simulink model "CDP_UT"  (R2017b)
settings: Solver=FixedStepDiscrete  StartTime=0.0  StopTime=10.0  FixedStep=0.01  RelTol=1e-3  EnableMultiTasking=on
undefined symbols (not defined in the file): ASWTYPE_FALSE, ASWTYPE_TRUE, CaCDP_CellTempNTCVoltTable_mV, CaCDP_CellTempTable_C, CaCDP_CMUPCBTempNTCVoltTable_mV, CaCDP_CMUPCBTempTable_C, CbCDP_DiffBusbarTempStateCheck_flg, CbCDP_DiffCellTempStateCheck_flg, CbCDP_DiffCellVoltStateCheck_flg, CbCDP_IgnorUpdateVld_flg, CbCDP_MaxBusbarTempStateCheck_flg, CbCDP_MaxCellTempStateCheck_flg, CbCDP_MaxCellVoltStateCheck_flg, CbCDP_MinBusbarTempStateCheck_flg, CbCDP_MinCellTempStateCheck_flg, CbCDP_MinCellVoltStateCheck_flg, CcCDP_AFETempConfig_numb, CcCDP_AFETempFltThd_C, CcCDP_AFETempFltThdHys_C, CcCDP_BusbarTempRngFltHiThrd_C, CcCDP_BusbarTempRngFltLowThrd_C, CcCDP_CellDiffFltLevel1_mV, CcCDP_CellDiffFltLevel2_mV, CcCDP_CellDiffFltLevel3_mV, CcCDP_CellTempLowerLimit_C, CcCDP_CellTempRngFltHiThrd_C, CcCDP_CellTempRngFltLowThrd_C, CcCDP_CellTempUpperLimit_C, CcCDP_CellVoltConfig_numb, CcCDP_CellVoltLowerLimit_mV, CcCDP_CellVoltRngHiThrd_mV, CcCDP_CellVoltRngLowThrd_mV, CcCDP_CellVoltUpdateThrd_numb, CcCDP_CellVoltUpperLimit_mV, CcCDP_ChrgMaxCellTempFltLv1Thrd_C, CcCDP_ChrgMaxCellTempFltLv2Thrd_C, CcCDP_ChrgMaxCellTempFltLv3Thrd_C, CcCDP_ChrgMaxCellTempReturnDiff_C, CcCDP_ChrgMinCellTempFltLv1Thrd_C, CcCDP_ChrgMinCellTempFltLv2Thrd_C, CcCDP_ChrgMinCellTempFltLv3Thrd_C, CcCDP_ChrgMinCellTempReturnDiff_C, CcCDP_CMUPCBTempConfig_numb, CcCDP_CMUPCBTempFltThd_C, CcCDP_CMUPCBTempFltThdHys_C, CcCDP_DiffBusbarTempFltLevel1Thrd_C, CcCDP_DiffBusbarTempFltLevel2Thrd_C, CcCDP_DiffBusbarTempReturnDifference_C, CcCDP_DiffCellTempFltLevel1Thrd_C, CcCDP_DiffCellTempFltLevel2Thrd_C, CcCDP_DiffCellTempReturnDifference_C, CcCDP_DiffCellVoltReturnDifference_mV, CcCDP_DiffVoltCheckMaxCellTempCondition_C, CcCDP_DiffVoltCheckMaxCellVoltCondition_mV, CcCDP_DiffVoltCheckMinCellTempCondition_C, CcCDP_DiffVoltCheckMinCellVoltCondition_mV, CcCDP_DiffVoltCheckPackCurrCondition_A, CcCDP_MaxAFETempIniVal_C, CcCDP_MaxBusbarTempFltLevel1Thrd_C, CcCDP_MaxBusbarTempFltLevel2Thrd_C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
libraries: AIWAYS_Powertrain_BMS_lib x148, simulink x8
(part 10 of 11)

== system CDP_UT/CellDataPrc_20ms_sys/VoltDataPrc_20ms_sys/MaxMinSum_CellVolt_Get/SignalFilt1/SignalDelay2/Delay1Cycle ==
  u : Inport
  Constant2 : Constant  Value=ASWTYPE_FALSE
  Switch : Switch  Criteria=u2 ~= 0  Threshold=1  RndMeth=Zero
  Unit Delay1 : UnitDelay  SampleTime=-1  StateName=StateName
  Unit Delay21 : UnitDelay  InitialCondition=1  SampleTime=-1  StateName=StateName
  y : Outport
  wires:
  Switch/1 -> y/1
  u/1 -> Switch/1, Unit Delay1/1
  Unit Delay1/1 -> Switch/3
  Unit Delay21/1 -> Switch/2
  Constant2/1 -> Unit Delay21/1

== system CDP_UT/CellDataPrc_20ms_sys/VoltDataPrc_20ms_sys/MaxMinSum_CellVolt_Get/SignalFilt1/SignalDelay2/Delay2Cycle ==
  u : Inport
  Constant2 : Constant  Value=ASWTYPE_FALSE
  Switch : Switch  Criteria=u2 ~= 0  Threshold=1  RndMeth=Zero
  Unit Delay1 : UnitDelay  SampleTime=-1  StateName=StateName
  Unit Delay2 : UnitDelay  InitialCondition=1  SampleTime=-1  StateName=StateName
  Unit Delay21 : UnitDelay  InitialCondition=1  SampleTime=-1  StateName=StateName
  Unit Delay3 : UnitDelay  SampleTime=-1  StateName=StateName
  y : Outport
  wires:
  Unit Delay3/1 -> Switch/3
  Unit Delay2/1 -> Switch/2
  Constant2/1 -> Unit Delay21/1
  Unit Delay21/1 -> Unit Delay2/1
  Unit Delay1/1 -> Unit Delay3/1
  u/1 -> Unit Delay1/1, Switch/1
  Switch/1 -> y/1

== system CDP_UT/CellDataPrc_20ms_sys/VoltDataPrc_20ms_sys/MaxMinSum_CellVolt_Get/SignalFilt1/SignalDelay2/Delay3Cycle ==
  u : Inport
  Constant2 : Constant  Value=ASWTYPE_FALSE
  Switch : Switch  Criteria=u2 ~= 0  Threshold=1  RndMeth=Zero
  Unit Delay1 : UnitDelay  SampleTime=-1  StateName=StateName
  Unit Delay2 : UnitDelay  InitialCondition=1  SampleTime=-1  StateName=StateName
  Unit Delay21 : UnitDelay  InitialCondition=1  SampleTime=-1  StateName=StateName
  Unit Delay3 : UnitDelay  SampleTime=-1  StateName=StateName
  Unit Delay4 : UnitDelay  InitialCondition=1  SampleTime=-1  StateName=StateName
  Unit Delay5 : UnitDelay  SampleTime=-1  StateName=StateName
  y : Outport
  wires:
  Unit Delay5/1 -> Switch/3
  Unit Delay4/1 -> Switch/2
  Unit Delay3/1 -> Unit Delay5/1
  Unit Delay2/1 -> Unit Delay4/1
  Constant2/1 -> Unit Delay21/1
  Unit Delay21/1 -> Unit Delay2/1
  Unit Delay1/1 -> Unit Delay3/1
  u/1 -> Unit Delay1/1, Switch/1
  Switch/1 -> y/1

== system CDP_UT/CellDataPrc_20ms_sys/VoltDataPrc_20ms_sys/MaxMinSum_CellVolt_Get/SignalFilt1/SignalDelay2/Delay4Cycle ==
  u : Inport
  Constant2 : Constant  Value=ASWTYPE_FALSE
  Switch : Switch  Criteria=u2 ~= 0  Threshold=1  RndMeth=Zero
  Unit Delay{1,3,5,7} (4 alike) : UnitDelay  SampleTime=-1  StateName=StateName
  Unit Delay{2,4,6,21} (4 alike) : UnitDelay  InitialCondition=1  SampleTime=-1  StateName=StateName
  y : Outport
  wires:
  Unit Delay7/1 -> Switch/3
  Unit Delay6/1 -> Switch/2
  Unit Delay5/1 -> Unit Delay7/1
  Unit Delay4/1 -> Unit Delay6/1
  Unit Delay3/1 -> Unit Delay5/1
  Unit Delay2/1 -> Unit Delay4/1
  Constant2/1 -> Unit Delay21/1
  Unit Delay21/1 -> Unit Delay2/1
  Unit Delay1/1 -> Unit Delay3/1
  u/1 -> Unit Delay1/1, Switch/1
  Switch/1 -> y/1

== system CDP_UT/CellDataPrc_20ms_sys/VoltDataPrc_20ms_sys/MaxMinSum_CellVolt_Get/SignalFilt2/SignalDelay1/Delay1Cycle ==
  u : Inport
  Constant2 : Constant  Value=ASWTYPE_FALSE
  Switch : Switch  Criteria=u2 ~= 0  Threshold=1  RndMeth=Zero
  Unit Delay1 : UnitDelay  SampleTime=-1  StateName=StateName
  Unit Delay21 : UnitDelay  InitialCondition=1  SampleTime=-1  StateName=StateName
  y : Outport
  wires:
  Constant2/1 -> Unit Delay21/1
  Unit Delay21/1 -> Switch/2
  Unit Delay1/1 -> Switch/3
  u/1 -> Unit Delay1/1, Switch/1
  Switch/1 -> y/1

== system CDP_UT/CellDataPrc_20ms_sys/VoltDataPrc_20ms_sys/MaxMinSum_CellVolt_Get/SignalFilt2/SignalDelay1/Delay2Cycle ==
  u : Inport
  Constant2 : Constant  Value=ASWTYPE_FALSE
  Switch : Switch  Criteria=u2 ~= 0  Threshold=1  RndMeth=Zero
  Unit Delay1 : UnitDelay  SampleTime=-1  StateName=StateName
  Unit Delay2 : UnitDelay  InitialCondition=1  SampleTime=-1  StateName=StateName
  Unit Delay21 : UnitDelay  InitialCondition=1  SampleTime=-1  StateName=StateName
  Unit Delay3 : UnitDelay  SampleTime=-1  StateName=StateName
  y : Outport
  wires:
  Switch/1 -> y/1
  u/1 -> Switch/1, Unit Delay1/1
  Unit Delay1/1 -> Unit Delay3/1
  Unit Delay21/1 -> Unit Delay2/1
  Constant2/1 -> Unit Delay21/1
  Unit Delay2/1 -> Switch/2
  Unit Delay3/1 -> Switch/3

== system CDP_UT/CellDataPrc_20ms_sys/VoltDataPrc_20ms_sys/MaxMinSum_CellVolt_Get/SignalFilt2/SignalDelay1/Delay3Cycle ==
  u : Inport
  Constant2 : Constant  Value=ASWTYPE_FALSE
  Switch : Switch  Criteria=u2 ~= 0  Threshold=1  RndMeth=Zero
  Unit Delay1 : UnitDelay  SampleTime=-1  StateName=StateName
  Unit Delay2 : UnitDelay  InitialCondition=1  SampleTime=-1  StateName=StateName
  Unit Delay21 : UnitDelay  InitialCondition=1  SampleTime=-1  StateName=StateName
  Unit Delay3 : UnitDelay  SampleTime=-1  StateName=StateName
  Unit Delay4 : UnitDelay  InitialCondition=1  SampleTime=-1  StateName=StateName
  Unit Delay5 : UnitDelay  SampleTime=-1  StateName=StateName
  y : Outport
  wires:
  Switch/1 -> y/1
  u/1 -> Switch/1, Unit Delay1/1
  Unit Delay1/1 -> Unit Delay3/1
  Unit Delay21/1 -> Unit Delay2/1
  Constant2/1 -> Unit Delay21/1
  Unit Delay2/1 -> Unit Delay4/1
  Unit Delay3/1 -> Unit Delay5/1
  Unit Delay4/1 -> Switch/2
  Unit Delay5/1 -> Switch/3

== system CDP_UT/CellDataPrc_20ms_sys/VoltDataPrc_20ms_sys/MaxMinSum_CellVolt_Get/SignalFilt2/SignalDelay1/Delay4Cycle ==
  u : Inport
  Constant2 : Constant  Value=ASWTYPE_FALSE
  Switch : Switch  Criteria=u2 ~= 0  Threshold=1  RndMeth=Zero
  Unit Delay{1,3,5,7} (4 alike) : UnitDelay  SampleTime=-1  StateName=StateName
  Unit Delay{2,4,6,21} (4 alike) : UnitDelay  InitialCondition=1  SampleTime=-1  StateName=StateName
  y : Outport
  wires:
  Switch/1 -> y/1
  u/1 -> Switch/1, Unit Delay1/1
  Unit Delay1/1 -> Unit Delay3/1
  Unit Delay21/1 -> Unit Delay2/1
  Constant2/1 -> Unit Delay21/1
  Unit Delay2/1 -> Unit Delay4/1
  Unit Delay3/1 -> Unit Delay5/1
  Unit Delay4/1 -> Unit Delay6/1
  Unit Delay5/1 -> Unit Delay7/1
  Unit Delay6/1 -> Switch/2
  Unit Delay7/1 -> Switch/3

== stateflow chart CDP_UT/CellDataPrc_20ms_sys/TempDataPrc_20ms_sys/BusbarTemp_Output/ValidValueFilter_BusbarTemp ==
  state VldValueFilter
    (default) -> (junction 1369)
    VldValueFilter -> (junction 1369)
    (junction 1369) -> (junction 1371) : {i = 0;}
    (junction 1373) -> (junction 1375) : [i < NumbConfig]
    (junction 1371) -> (junction 1373) : [i < InputNumb]
    (junction 1373) -> (junction 1377) : {OutputValue[i] = CcCDP_TempDefVal_C;}
    (junction 1375) -> (junction 1380) : {OutputValue[i] = InputValue[i];}
    (junction 1377) -> (junction 1371) : {i = i + 1;}
    (junction 1371) -> (junction 1385)
    (junction 1380) -> (junction 1377)
  (default) -> VldValueFilter
  data: InputValue input single; NumbConfig input uint8; i local uint8; CcCDP_TempDefVal_C parameter; OutputValue output single; InputNumb input uint8

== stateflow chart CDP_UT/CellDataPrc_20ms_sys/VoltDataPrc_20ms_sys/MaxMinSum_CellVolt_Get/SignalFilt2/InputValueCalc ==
  state VldValueFilter
    state Default
      Output_Value[0] = Input_Value;
      Output_Value[1] = Input_Value;
      Output_Value[2] = Input_Value;
      Output_Value[3] = Input_Value;
      Output_Value[4] = Input_Value;
    state NotUpdate
      Output_Value[0] = Old_Value[0];
      Output_Value[1] = Old_Value[1];
      Output_Value[2] = Old_Value[2];
      Output_Value[3] = Old_Value[3];
      Output_Value[4] = Old_Value[4];
    state Update
      Output_Value[0] = Input_Value;
      Output_Value[1] = Old_Value[0];
      Output_Value[2] = Old_Value[1];
      Output_Value[3] = Old_Value[2];
      Output_Value[4] = Old_Value[3];
    (default) -> Default
    VldValueFilter -> (junction 1397)
    (junction 1397) -> (junction 1398) : [Rige]
    (junction 1397) -> NotUpdate
    (junction 1398) -> Update
  (default) -> VldValueFilter
  data: Input_Value input uint16; Rige input boolean; Output_Value output uint16; Old_Value input uint16

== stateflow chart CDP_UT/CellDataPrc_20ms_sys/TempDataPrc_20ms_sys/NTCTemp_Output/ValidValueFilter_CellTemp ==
  state VldValueFilter
    (default) -> (junction 1369)
    VldValueFilter -> (junction 1369)
    (junction 1369) -> (junction 1371) : {i = 0;}
    (junction 1373) -> (junction 1375) : [i < NumbConfig]
    (junction 1371) -> (junction 1373) : [i < InputNumb]
    (junction 1373) -> (junction 1377) : {OutputValue[i] = CcCDP_TempDefVal_C;}
    (junction 1375) -> (junction 1380) : {OutputValue[i] = InputValue[i];}
    (junction 1377) -> (junction 1371) : {i = i + 1;}
    (junction 1371) -> (junction 1385)
    (junction 1380) -> (junction 1377)
  (default) -> VldValueFilter
  data: InputValue input single; NumbConfig input uint8; i local uint8; CcCDP_TempDefVal_C parameter; OutputValue output single; InputNumb input uint8

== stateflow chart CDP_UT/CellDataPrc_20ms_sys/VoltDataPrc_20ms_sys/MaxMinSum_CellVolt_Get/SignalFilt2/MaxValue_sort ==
  state sort
    (default) -> (junction 6) : /*Input value sort from big to small*/
    sort -> (junction 6)
    (junction 6) -> (junction 8) : {i = 0;temp = 0;}
    (junction 8) -> (junction 12) : [i < Input_dim]
    (junction 12) -> (junction 14) : {Output_Value[i] = Input_Value[i];}
    (junction 14) -> (junction 8) : {i++;}
    (junction 8) -> (junction 17) : {i=0;}
    (junction 25) -> (junction 31) : [Output_Value[j] > temp]
    (junction 17) -> (junction 19) : [i < Input_dim]
    (junction 21) -> (junction 25) : [j < Input_dim]
    (junction 19) -> (junction 21) : {temp = 0;Output_index[i] = 0;j = 0;}
    (junction 25) -> (junction 34)
    (junction 31) -> (junction 32) : {temp = Output_Value[j]; Output_index[i] = j;}
    (junction 38) -> (junction 17) : {i++;}
    (junction 34) -> (junction 21) : {j++;}
    (junction 21) -> (junction 38) : {Output_Value[Output_index[i]] = 0;}
    (junction 17) -> (junction 41) : {i= 0;}
    (junction 32) -> (junction 34)
    (junction 41) -> (junction 43) : [i < Input_dim]
    (junction 43) -> (junction 45) : {Output_Value[i] = Input_Value[Output_index[i]];}
    (junction 45) -> (junction 41) : {i++;}
    (junction 41) -> (junction 48)
  (default) -> sort
  data: Input_Value input uint16; Input_dim input uint8; Output_Value output single; i local uint8; temp local single; j local uint8; Output_index output uint16

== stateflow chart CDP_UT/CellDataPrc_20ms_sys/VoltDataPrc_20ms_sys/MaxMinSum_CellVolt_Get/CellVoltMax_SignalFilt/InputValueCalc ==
  state VldValueFilter
    state Default
      Output_Value[0] = Input_Value;
      Output_Value[1] = Input_Value;
      Output_Value[2] = Input_Value;
      Output_Value[3] = Input_Value;
      Output_Value[4] = Input_Value;
    state NotUpdate
      Output_Value[0] = Old_Value[0];
      Output_Value[1] = Old_Value[1];
      Output_Value[2] = Old_Value[2];
      Output_Value[3] = Old_Value[3];
      Output_Value[4] = Old_Value[4];
    state Update
      Output_Value[0] = Input_Value;
      Output_Value[1] = Old_Value[0];
      Output_Value[2] = Old_Value[1];
      Output_Value[3] = Old_Value[2];
      Output_Value[4] = Old_Value[3];
    (default) -> Default
    VldValueFilter -> (junction 1397)
    (junction 1397) -> (junction 1398) : [Rige]
    (junction 1397) -> NotUpdate
    (junction 1398) -> Update
  (default) -> VldValueFilter
  data: Input_Value input uint16; Rige input boolean; Output_Value output uint16; Old_Value input uint16

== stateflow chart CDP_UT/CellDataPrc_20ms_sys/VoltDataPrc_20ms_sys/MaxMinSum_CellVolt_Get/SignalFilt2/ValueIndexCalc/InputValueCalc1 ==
  state VldValueFilter
    state Default
      Output_Value[0] = Input_Value;
      Output_Value[1] = Input_Value;
      Output_Value[2] = Input_Value;
      Output_Value[3] = Input_Value;
      Output_Value[4] = Input_Value;
    state NotUpdate
      Output_Value[0] = Old_Value[0];
      Output_Value[1] = Old_Value[1];
      Output_Value[2] = Old_Value[2];
      Output_Value[3] = Old_Value[3];
      Output_Value[4] = Old_Value[4];
    state Update
      Output_Value[0] = Input_Value;
      Output_Value[1] = Old_Value[0];
      Output_Value[2] = Old_Value[1];
      Output_Value[3] = Old_Value[2];
      Output_Value[4] = Old_Value[3];
    (default) -> Default
    VldValueFilter -> (junction 1397)
    (junction 1397) -> (junction 1398) : [Rige]
    (junction 1397) -> NotUpdate
    (junction 1398) -> Update
  (default) -> VldValueFilter
  data: Input_Value input uint16; Rige input boolean; Output_Value output uint16; Old_Value input uint16

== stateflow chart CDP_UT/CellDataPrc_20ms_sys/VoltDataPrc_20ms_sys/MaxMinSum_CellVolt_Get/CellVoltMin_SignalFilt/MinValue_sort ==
  state sort
    (default) -> (junction 1403) : /*Input value sort from big to small*/
    sort -> (junction 1403)
    (junction 1403) -> (junction 1442) : {i = 0;temp = 0;}
    (junction 1442) -> (junction 1433) : [i < Input_dim]
    (junction 1433) -> (junction 1413) : {Output_Value[i] = Input_Value[i];}
    (junction 1413) -> (junction 1442) : {i++;}
    (junction 1442) -> (junction 1431) : {i=0;}
    (junction 1425) -> (junction 1421) : [Output_Value[j] > temp]
    (junction 1431) -> (junction 1430) : [i < Input_dim]
    (junction 1437) -> (junction 1425) : [j < Input_dim]
    (junction 1430) -> (junction 1437) : {temp = 0;Output_index[i] = 0;j = 0;}
    (junction 1425) -> (junction 1404)
    (junction 1421) -> (junction 1418) : {temp = Output_Value[j]; Output_index[i] = j;}
    (junction 1435) -> (junction 1431) : {i++;}
    (junction 1404) -> (junction 1437) : {j++;}
    (junction 1437) -> (junction 1435) : {Output_Value[Output_index[i]] = 0;}
    (junction 1431) -> (junction 1420) : {i= 0;}
    (junction 1418) -> (junction 1404)
    (junction 1420) -> (junction 1426) : [i < Input_dim]
    (junction 1426) -> (junction 1429) : {Output_Value[i] = Input_Value[Output_index[i]];}
    (junction 1429) -> (junction 1420) : {i++;}
    (junction 1420) -> (junction 1438)
  (default) -> sort
  data: Input_Value input uint16; Output_Value output uint16; Input_dim input uint8; Output_index output uint8; i local uint8; j local uint8; temp local uint16

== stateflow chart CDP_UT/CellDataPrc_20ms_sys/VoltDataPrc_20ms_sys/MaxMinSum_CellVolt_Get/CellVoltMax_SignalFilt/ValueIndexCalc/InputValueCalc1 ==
  state VldValueFilter
    state Default
      Output_Value[0] = Input_Value;
      Output_Value[1] = Input_Value;
      Output_Value[2] = Input_Value;
      Output_Value[3] = Input_Value;
      Output_Value[4] = Input_Value;
    state NotUpdate
      Output_Value[0] = Old_Value[0];
      Output_Value[1] = Old_Value[1];
      Output_Value[2] = Old_Value[2];
      Output_Value[3] = Old_Value[3];
      Output_Value[4] = Old_Value[4];
    state Update
      Output_Value[0] = Input_Value;
      Output_Value[1] = Old_Value[0];
      Output_Value[2] = Old_Value[1];
      Output_Value[3] = Old_Value[2];
      Output_Value[4] = Old_Value[3];
    (default) -> Default
    VldValueFilter -> (junction 1397)
    (junction 1397) -> (junction 1398) : [Rige]
    (junction 1397) -> NotUpdate
    (junction 1398) -> Update
  (default) -> VldValueFilter
  data: Input_Value input uint8; Rige input boolean; Output_Value output uint8; Old_Value input uint8

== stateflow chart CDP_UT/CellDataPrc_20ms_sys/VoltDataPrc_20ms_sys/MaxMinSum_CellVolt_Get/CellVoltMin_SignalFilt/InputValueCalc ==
  state VldValueFilter
    state Default
      Output_Value[0] = Input_Value;
      Output_Value[1] = Input_Value;
      Output_Value[2] = Input_Value;
      Output_Value[3] = Input_Value;
      Output_Value[4] = Input_Value;
    state NotUpdate
      Output_Value[0] = Old_Value[0];
      Output_Value[1] = Old_Value[1];
      Output_Value[2] = Old_Value[2];
      Output_Value[3] = Old_Value[3];
      Output_Value[4] = Old_Value[4];
    state Update
      Output_Value[0] = Input_Value;
      Output_Value[1] = Old_Value[0];
      Output_Value[2] = Old_Value[1];
      Output_Value[3] = Old_Value[2];
      Output_Value[4] = Old_Value[3];
    (default) -> Default
    VldValueFilter -> (junction 1397)
    (junction 1397) -> (junction 1398) : [Rige]
    (junction 1397) -> NotUpdate
    (junction 1398) -> Update
  (default) -> VldValueFilter
  data: Input_Value input uint16; Rige input boolean; Output_Value output uint16; Old_Value input uint16

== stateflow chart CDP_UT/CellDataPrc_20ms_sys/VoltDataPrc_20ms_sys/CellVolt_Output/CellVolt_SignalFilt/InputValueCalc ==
  state Default
    (default) -> (junction 1481) : %{Output_Value[0] = Input_Value; %Output_Value[1] = Input_Value; %Output_Value[2] = Input_Value; %Output_Value[3] = Input_Value; %Output_Value[4] = Input_Value;}
    (junction 1481) -> (junction 1483) : {i = 0;}
    (junction 1483) -> (junction 1485) : [i <Input_num]
    (junction 1485) -> (junction 1487) : {Output_Value[0][i] = Input_Value[i]; Output_Value[1][i] = Input_Value[i]; Output_Value[2][i] = Input_Value[i]; Output_Value[3][i] = Input_Value[i]; Output_Value[4][i] = Input_Value[i];}
    (junction 1487) -> (junction 1483) : {i++;}
    (junction 1483) -> (junction 1490)
  state Update
    (default) -> (junction 1458)
    (junction 1458) -> (junction 1461) : {i = 0;}
    Update -> (junction 1461)
    (junction 1461) -> (junction 1463) : [i < Input_num]
    (junction 1463) -> (junction 1465) : [Update[i]]
    (junction 1469) -> (junction 1461) : {i++;}
    (junction 1461) -> (junction 1476) : {i = 0;}
    (junction 1463) -> (junction 1469) : {Output_Value[0][i] = Old_Value[0][i]; Output_Value[1][i] = Old_Value[1][i]; Output_Value[2][i] = Old_Value[2][i]; Output_Value[3][i] = Old_Value[3][i]; Output_Value[4][i] = Old_Value[4][i];}
    (junction 1465) -> (junction 1467) : {Output_Value[0][i] = Input_Value[i]; Output_Value[1][i] = Old_Value[0][i]; Output_Value[2][i] = Old_Value[1][i]; Output_Value[3][i] = Old_Value[2][i]; Output_Value[4][i] = Old_Value[3][i];}
    (junction 1467) -> (junction 1469)
  (default) -> Default
  Default -> Update : [i >Input_num-1]
  data: Input_Value input uint16; Update input boolean; Output_Value output uint16; i local uint8; Input_num input uint8; Old_Value input uint16

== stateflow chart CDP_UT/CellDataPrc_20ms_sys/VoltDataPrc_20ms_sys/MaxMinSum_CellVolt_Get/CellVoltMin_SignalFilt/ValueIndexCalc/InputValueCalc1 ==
  state VldValueFilter
    state Default
      Output_Value[0] = Input_Value;
      Output_Value[1] = Input_Value;
      Output_Value[2] = Input_Value;
      Output_Value[3] = Input_Value;
      Output_Value[4] = Input_Value;
    state NotUpdate
      Output_Value[0] = Old_Value[0];
      Output_Value[1] = Old_Value[1];
      Output_Value[2] = Old_Value[2];
      Output_Value[3] = Old_Value[3];
      Output_Value[4] = Old_Value[4];
    state Update
      Output_Value[0] = Input_Value;
      Output_Value[1] = Old_Value[0];
      Output_Value[2] = Old_Value[1];
      Output_Value[3] = Old_Value[2];
      Output_Value[4] = Old_Value[3];
    (default) -> Default
    VldValueFilter -> (junction 1397)
    (junction 1397) -> (junction 1398) : [Rige]
    (junction 1397) -> NotUpdate
    (junction 1398) -> Update
  (default) -> VldValueFilter
  data: Input_Value input uint8; Rige input boolean; Output_Value output uint8; Old_Value input uint8

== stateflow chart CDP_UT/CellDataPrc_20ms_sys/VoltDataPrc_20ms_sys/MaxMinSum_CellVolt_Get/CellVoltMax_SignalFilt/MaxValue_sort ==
  state sort
    (default) -> (junction 1403) : /*Input value sort from big to small*/
    sort -> (junction 1403)
    (junction 1403) -> (junction 1442) : {i = 0;temp = 0;}
    (junction 1442) -> (junction 1433) : [i < Input_dim]
    (junction 1433) -> (junction 1413) : {Output_Value[i] = Input_Value[i];}
    (junction 1413) -> (junction 1442) : {i++;}
    (junction 1442) -> (junction 1431) : {i=0;}
    (junction 1425) -> (junction 1421) : [Output_Value[j] > temp]
    (junction 1431) -> (junction 1430) : [i < Input_dim]
    (junction 1437) -> (junction 1425) : [j < Input_dim]
    (junction 1430) -> (junction 1437) : {temp = 0;Output_index[i] = 0;j = 0;}
    (junction 1425) -> (junction 1404)
    (junction 1421) -> (junction 1418) : {temp = Output_Value[j]; Output_index[i] = j;}
    (junction 1435) -> (junction 1431) : {i++;}
    (junction 1404) -> (junction 1437) : {j++;}
    (junction 1437) -> (junction 1435) : {Output_Value[Output_index[i]] = 0;}
    (junction 1431) -> (junction 1420) : {i= 0;}
    (junction 1418) -> (junction 1404)
    (junction 1420) -> (junction 1426) : [i < Input_dim]
    (junction 1426) -> (junction 1429) : {Output_Value[i] = Input_Value[Output_index[i]];}
    (junction 1429) -> (junction 1420) : {i++;}
    (junction 1420) -> (junction 1438)
  (default) -> sort
  data: Input_Value input uint16; Output_Value output uint16; Input_dim input uint8; Output_index output uint8; i local uint8; j local uint8; temp local uint16

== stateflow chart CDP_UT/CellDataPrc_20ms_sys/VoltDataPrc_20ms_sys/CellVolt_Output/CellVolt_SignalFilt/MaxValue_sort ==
  state sort
    (default) -> (junction 1403) : /*Input value sort from big to small*/
    sort -> (junction 1403)
    (junction 1403) -> (junction 1442) : {i = 0;j = 0;}
    (junction 1433) -> (junction 1448) : [j < Input_num]
    (junction 1442) -> (junction 1433) : [i < Input_dim]
    (junction 1450) -> (junction 1433) : {j++;}
    (junction 1433) -> (junction 1413)
    (junction 1448) -> (junction 1450) : {Output_Value[i][j] = Input_Value[i][j];}
    (junction 1413) -> (junction 1442) : {i++;j=0;}
    (junction 1442) -> (junction 1509)
    (junction 1509) -> (junction 1508) : [Input_dim == 1]
    (junction 1509) -> (junction 1431) : {m=Input_dim -1;n = 3;k = 0;}
    (junction 1508) -> (junction 1512)
    (junction 1430) -> (junction 1437) : {temp = 0;n = m-1;}
    (junction 1437) -> (junction 1488) : [n>=0]
    (junction 1488) -> (junction 1474) : [Output_Value[n][k] > Output_Value[m][k]]
    (junction 1454) -> (junction 1430) : [m >= 1]
    (junction 1492) -> (junction 1437) : {n--;}
    (junction 1437) -> (junction 1485)
    (junction 1488) -> (junction 1492)
    (junction 1474) -> (junction 1476) : {temp=Output_Value[n][k]; Output_Value[n][k]=Output_Value[m][k]; Output_Value[m][k]=temp;}
    (junction 1431) -> (junction 1455) : [k<Input_num]
    (junction 1455) -> (junction 1454)
    (junction 1459) -> (junction 1431) : {k++;m=Input_dim -1;}
    (junction 1431) -> (junction 1420)
    (junction 1435) -> (junction 1454) : {m=m-1;}
    (junction 1454) -> (junction 1459)
    (junction 1485) -> (junction 1435)
    (junction 1476) -> (junction 1492)
    (junction 1512) -> (junction 1420)
    (junction 1420) -> (junction 1497) : {h = (Input_dim - 1)/2; k=0;}
    (junction 1497) -> (junction 1499) : [k<Input_num]
    (junction 1499) -> (junction 1501) : {TargetOutput_Value[k] = Output_Value[h][k];}
    (junction 1501) -> (junction 1497) : {k++;}
    (junction 1497) -> (junction 1504)
  (default) -> sort
  data: Input_Value input uint16; Output_Value output uint16; Input_dim input uint8; i local uint8; j local uint8; temp local uint16; k local uint8; n local int8; m local uint8; TargetOutput_Value output uint16; h local uint8; Input_num input uint8

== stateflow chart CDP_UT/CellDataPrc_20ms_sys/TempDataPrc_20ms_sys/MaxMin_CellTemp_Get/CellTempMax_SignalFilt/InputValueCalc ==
  state VldValueFilter
    state Default
      Output_Value[0] = Input_Value;
      Output_Value[1] = Input_Value;
      Output_Value[2] = Input_Value;
      Output_Value[3] = Input_Value;
      Output_Value[4] = Input_Value;
    state NotUpdate
      Output_Value[0] = Old_Value[0];
      Output_Value[1] = Old_Value[1];
      Output_Value[2] = Old_Value[2];
      Output_Value[3] = Old_Value[3];
      Output_Value[4] = Old_Value[4];
    state Update
      Output_Value[0] = Input_Value;
      Output_Value[1] = Old_Value[0];
      Output_Value[2] = Old_Value[1];
      Output_Value[3] = Old_Value[2];
      Output_Value[4] = Old_Value[3];
    (default) -> Default
    VldValueFilter -> (junction 1397)
    (junction 1397) -> (junction 1398) : [Rige]
    (junction 1397) -> NotUpdate
    (junction 1398) -> Update
  (default) -> VldValueFilter
  data: Input_Value input single; Rige input boolean; Output_Value output single; Old_Value input single

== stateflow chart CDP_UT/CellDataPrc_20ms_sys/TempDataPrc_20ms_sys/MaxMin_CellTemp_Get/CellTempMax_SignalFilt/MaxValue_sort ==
  state sort
    (default) -> (junction 1403) : /*Input value sort from big to small*/
    sort -> (junction 1403)
    (junction 1403) -> (junction 1442) : {i = 0;temp = 0;}
    (junction 1442) -> (junction 1433) : [i < Input_dim]
    (junction 1433) -> (junction 1413) : {Output_Value[i] = Input_Value[i];}
    (junction 1413) -> (junction 1442) : {i++;}
    (junction 1442) -> (junction 1431) : {i=0;}
    (junction 1425) -> (junction 1421) : [Output_Value[j] > temp]
    (junction 1431) -> (junction 1430) : [i < Input_dim]
    (junction 1437) -> (junction 1425) : [j < Input_dim]
    (junction 1430) -> (junction 1437) : {temp = 0;Output_index[i] = 0;j = 0;}
    (junction 1425) -> (junction 1404)
    (junction 1421) -> (junction 1418) : {temp = Output_Value[j]; Output_index[i] = j;}
    (junction 1435) -> (junction 1431) : {i++;}
    (junction 1404) -> (junction 1437) : {j++;}
    (junction 1437) -> (junction 1435) : {Output_Value[Output_index[i]] = 0;}
    (junction 1431) -> (junction 1420) : {i= 0;}
    (junction 1418) -> (junction 1404)
    (junction 1420) -> (junction 1426) : [i < Input_dim]
    (junction 1426) -> (junction 1429) : {Output_Value[i] = Input_Value[Output_index[i]];}
    (junction 1429) -> (junction 1420) : {i++;}
    (junction 1420) -> (junction 1438)
  (default) -> sort
  data: Input_Value input single; Output_Value output single; Input_dim input uint8; Output_index output uint8; i local uint8; j local uint8; temp local single

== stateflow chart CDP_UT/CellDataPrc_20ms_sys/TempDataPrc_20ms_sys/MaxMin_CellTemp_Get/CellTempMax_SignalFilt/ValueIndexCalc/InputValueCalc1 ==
  state VldValueFilter
    state Default
      Output_Value[0] = Input_Value;
      Output_Value[1] = Input_Value;
      Output_Value[2] = Input_Value;
      Output_Value[3] = Input_Value;
      Output_Value[4] = Input_Value;
    state NotUpdate
      Output_Value[0] = Old_Value[0];
      Output_Value[1] = Old_Value[1];
      Output_Value[2] = Old_Value[2];
      Output_Value[3] = Old_Value[3];
      Output_Value[4] = Old_Value[4];
    state Update
      Output_Value[0] = Input_Value;
      Output_Value[1] = Old_Value[0];
      Output_Value[2] = Old_Value[1];
      Output_Value[3] = Old_Value[2];
      Output_Value[4] = Old_Value[3];
    (default) -> Default
    VldValueFilter -> (junction 1397)
    (junction 1397) -> (junction 1398) : [Rige]
    (junction 1397) -> NotUpdate
    (junction 1398) -> Update
  (default) -> VldValueFilter
  data: Input_Value input uint8; Rige input boolean; Output_Value output uint8; Old_Value input uint8

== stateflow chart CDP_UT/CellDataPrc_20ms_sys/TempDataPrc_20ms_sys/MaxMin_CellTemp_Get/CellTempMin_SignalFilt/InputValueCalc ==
  state VldValueFilter
    state Default
      Output_Value[0] = Input_Value;
      Output_Value[1] = Input_Value;
      Output_Value[2] = Input_Value;
      Output_Value[3] = Input_Value;
      Output_Value[4] = Input_Value;
    state NotUpdate
      Output_Value[0] = Old_Value[0];
      Output_Value[1] = Old_Value[1];
      Output_Value[2] = Old_Value[2];
      Output_Value[3] = Old_Value[3];
      Output_Value[4] = Old_Value[4];
    state Update
      Output_Value[0] = Input_Value;
      Output_Value[1] = Old_Value[0];
      Output_Value[2] = Old_Value[1];
      Output_Value[3] = Old_Value[2];
      Output_Value[4] = Old_Value[3];
    (default) -> Default
    VldValueFilter -> (junction 1397)
    (junction 1397) -> (junction 1398) : [Rige]
    (junction 1397) -> NotUpdate
    (junction 1398) -> Update
  (default) -> VldValueFilter
  data: Input_Value input single; Rige input boolean; Output_Value output single; Old_Value input single

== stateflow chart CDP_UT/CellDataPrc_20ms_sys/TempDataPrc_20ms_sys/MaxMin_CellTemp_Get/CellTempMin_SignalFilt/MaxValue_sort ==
  state sort
    (default) -> (junction 1403) : /*Input value sort from big to small*/
    sort -> (junction 1403)
    (junction 1403) -> (junction 1442) : {i = 0;temp = 0;}
    (junction 1442) -> (junction 1433) : [i < Input_dim]
    (junction 1433) -> (junction 1413) : {Output_Value[i] = Input_Value[i];}
    (junction 1413) -> (junction 1442) : {i++;}
    (junction 1442) -> (junction 1431) : {i=0;}
    (junction 1425) -> (junction 1421) : [Output_Value[j] > temp]
    (junction 1431) -> (junction 1430) : [i < Input_dim]
    (junction 1437) -> (junction 1425) : [j < Input_dim]
    (junction 1430) -> (junction 1437) : {temp = 0;Output_index[i] = 0;j = 0;}
    (junction 1425) -> (junction 1404)
    (junction 1421) -> (junction 1418) : {temp = Output_Value[j]; Output_index[i] = j;}
    (junction 1435) -> (junction 1431) : {i++;}
    (junction 1404) -> (junction 1437) : {j++;}
    (junction 1437) -> (junction 1435) : {Output_Value[Output_index[i]] = 0;}
    (junction 1431) -> (junction 1420) : {i= 0;}
    (junction 1418) -> (junction 1404)
    (junction 1420) -> (junction 1426) : [i < Input_dim]
    (junction 1426) -> (junction 1429) : {Output_Value[i] = Input_Value[Output_index[i]];}
    (junction 1429) -> (junction 1420) : {i++;}
    (junction 1420) -> (junction 1438)
  (default) -> sort
  data: Input_Value input single; Output_Value output single; Input_dim input uint8; Output_index output uint8; i local uint8; j local uint8; temp local single

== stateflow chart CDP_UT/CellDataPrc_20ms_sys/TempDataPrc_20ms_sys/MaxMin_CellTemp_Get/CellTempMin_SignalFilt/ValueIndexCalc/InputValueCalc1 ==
  state VldValueFilter
    state Default
      Output_Value[0] = Input_Value;
      Output_Value[1] = Input_Value;
      Output_Value[2] = Input_Value;
      Output_Value[3] = Input_Value;
      Output_Value[4] = Input_Value;
    state NotUpdate
      Output_Value[0] = Old_Value[0];
      Output_Value[1] = Old_Value[1];
      Output_Value[2] = Old_Value[2];
      Output_Value[3] = Old_Value[3];
      Output_Value[4] = Old_Value[4];
    state Update
      Output_Value[0] = Input_Value;
      Output_Value[1] = Old_Value[0];
      Output_Value[2] = Old_Value[1];
      Output_Value[3] = Old_Value[2];
      Output_Value[4] = Old_Value[3];
    (default) -> Default
    VldValueFilter -> (junction 1397)
    (junction 1397) -> (junction 1398) : [Rige]
    (junction 1397) -> NotUpdate
    (junction 1398) -> Update
  (default) -> VldValueFilter
  data: Input_Value input uint8; Rige input boolean; Output_Value output uint8; Old_Value input uint8

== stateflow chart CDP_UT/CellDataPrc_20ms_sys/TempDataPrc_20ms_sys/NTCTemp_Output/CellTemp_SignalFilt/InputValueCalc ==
  state Default
    (default) -> (junction 1481) : %{Output_Value[0] = Input_Value; %Output_Value[1] = Input_Value; %Output_Value[2] = Input_Value; %Output_Value[3] = Input_Value; %Output_Value[4] = Input_Value;}
    (junction 1481) -> (junction 1483) : {i = 0;}
    (junction 1483) -> (junction 1485) : [i <Input_num]
    (junction 1485) -> (junction 1487) : {Output_Value[0][i] = Input_Value[i]; Output_Value[1][i] = Input_Value[i]; Output_Value[2][i] = Input_Value[i]; Output_Value[3][i] = Input_Value[i]; Output_Value[4][i] = Input_Value[i];}
    (junction 1487) -> (junction 1483) : {i++;}
    (junction 1483) -> (junction 1490)
  state Update
    (default) -> (junction 1458)
    (junction 1458) -> (junction 1461) : {i = 0;}
    Update -> (junction 1461)
    (junction 1461) -> (junction 1463) : [i < Input_num]
    (junction 1463) -> (junction 1465) : [Update[i]]
    (junction 1469) -> (junction 1461) : {i++;}
    (junction 1461) -> (junction 1476) : {i = 0;}
    (junction 1463) -> (junction 1469) : {Output_Value[0][i] = Old_Value[0][i]; Output_Value[1][i] = Old_Value[1][i]; Output_Value[2][i] = Old_Value[2][i]; Output_Value[3][i] = Old_Value[3][i]; Output_Value[4][i] = Old_Value[4][i];}
    (junction 1465) -> (junction 1467) : {Output_Value[0][i] = Input_Value[i]; Output_Value[1][i] = Old_Value[0][i]; Output_Value[2][i] = Old_Value[1][i]; Output_Value[3][i] = Old_Value[2][i]; Output_Value[4][i] = Old_Value[3][i];}
    (junction 1467) -> (junction 1469)
  (default) -> Default
  Default -> Update : [i >Input_num-1]
  data: Input_Value input single; Update input boolean; Output_Value output single; i local uint8; Input_num input uint8; Old_Value input single

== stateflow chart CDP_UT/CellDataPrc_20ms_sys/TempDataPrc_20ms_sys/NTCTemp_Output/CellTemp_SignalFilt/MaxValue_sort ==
  state sort
    (default) -> (junction 1403) : /*Input value sort from big to small*/
    sort -> (junction 1403)
    (junction 1403) -> (junction 1442) : {i = 0;j = 0;}
    (junction 1433) -> (junction 1448) : [j < Input_num]
    (junction 1442) -> (junction 1433) : [i < Input_dim]
    (junction 1450) -> (junction 1433) : {j++;}
    (junction 1433) -> (junction 1413)
    (junction 1448) -> (junction 1450) : {Output_Value[i][j] = Input_Value[i][j];}
    (junction 1413) -> (junction 1442) : {i++;j=0;}
    (junction 1442) -> (junction 1509)
    (junction 1509) -> (junction 1508) : [Input_dim == 1]
    (junction 1509) -> (junction 1431) : {m=Input_dim -1;n = 3;k = 0;}
    (junction 1508) -> (junction 1512)
    (junction 1430) -> (junction 1437) : {temp = 0;n = m-1;}
    (junction 1437) -> (junction 1488) : [n>=0]
    (junction 1488) -> (junction 1474) : [Output_Value[n][k] > Output_Value[m][k]]
    (junction 1454) -> (junction 1430) : [m >= 1]
    (junction 1492) -> (junction 1437) : {n--;}
    (junction 1437) -> (junction 1485)
    (junction 1488) -> (junction 1492)
    (junction 1474) -> (junction 1476) : {temp=Output_Value[n][k]; Output_Value[n][k]=Output_Value[m][k]; Output_Value[m][k]=temp;}
    (junction 1431) -> (junction 1455) : [k<Input_num]
    (junction 1455) -> (junction 1454)
    (junction 1459) -> (junction 1431) : {k++;m=Input_dim -1;}
    (junction 1431) -> (junction 1420)
    (junction 1435) -> (junction 1454) : {m=m-1;}
    (junction 1454) -> (junction 1459)
    (junction 1485) -> (junction 1435)
    (junction 1476) -> (junction 1492)
    (junction 1512) -> (junction 1420)
    (junction 1420) -> (junction 1497) : {h = (Input_dim - 1)/2; k=0;}
    (junction 1497) -> (junction 1499) : [k<Input_num]
    (junction 1499) -> (junction 1501) : {TargetOutput_Value[k] = Output_Value[h][k];}
    (junction 1501) -> (junction 1497) : {k++;}
    (junction 1497) -> (junction 1504)
  (default) -> sort
  data: Input_Value input single; Output_Value output single; Input_dim input uint8; i local uint8; j local uint8; temp local single; k local uint8; n local int8; m local uint8; TargetOutput_Value output single; h local uint8; Input_num input uint8

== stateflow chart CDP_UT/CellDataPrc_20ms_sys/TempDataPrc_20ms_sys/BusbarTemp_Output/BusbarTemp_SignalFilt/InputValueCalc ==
  state Default
    (default) -> (junction 1481) : %{Output_Value[0] = Input_Value; %Output_Value[1] = Input_Value; %Output_Value[2] = Input_Value; %Output_Value[3] = Input_Value; %Output_Value[4] = Input_Value;}
    (junction 1481) -> (junction 1483) : {i = 0;}
    (junction 1483) -> (junction 1485) : [i <Input_num]
    (junction 1485) -> (junction 1487) : {Output_Value[0][i] = Input_Value[i]; Output_Value[1][i] = Input_Value[i]; Output_Value[2][i] = Input_Value[i]; Output_Value[3][i] = Input_Value[i]; Output_Value[4][i] = Input_Value[i];}
    (junction 1487) -> (junction 1483) : {i++;}
    (junction 1483) -> (junction 1490)
  state Update
    (default) -> (junction 1458)
    (junction 1458) -> (junction 1461) : {i = 0;}
    Update -> (junction 1461)
    (junction 1461) -> (junction 1463) : [i < Input_num]
    (junction 1463) -> (junction 1465) : [Update[i]]
    (junction 1469) -> (junction 1461) : {i++;}
    (junction 1461) -> (junction 1476) : {i = 0;}
    (junction 1463) -> (junction 1469) : {Output_Value[0][i] = Old_Value[0][i]; Output_Value[1][i] = Old_Value[1][i]; Output_Value[2][i] = Old_Value[2][i]; Output_Value[3][i] = Old_Value[3][i]; Output_Value[4][i] = Old_Value[4][i];}
    (junction 1465) -> (junction 1467) : {Output_Value[0][i] = Input_Value[i]; Output_Value[1][i] = Old_Value[0][i]; Output_Value[2][i] = Old_Value[1][i]; Output_Value[3][i] = Old_Value[2][i]; Output_Value[4][i] = Old_Value[3][i];}
    (junction 1467) -> (junction 1469)
  (default) -> Default
  Default -> Update : [i >Input_num-1]
  data: Input_Value input single; Update input boolean; Output_Value output single; i local uint8; Input_num input uint8; Old_Value input single

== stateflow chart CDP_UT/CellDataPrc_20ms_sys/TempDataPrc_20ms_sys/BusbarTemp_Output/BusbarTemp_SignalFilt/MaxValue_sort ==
  state sort
    (default) -> (junction 1403) : /*Input value sort from big to small*/
    sort -> (junction 1403)
    (junction 1403) -> (junction 1442) : {i = 0;j = 0;}
    (junction 1433) -> (junction 1448) : [j < Input_num]
    (junction 1442) -> (junction 1433) : [i < Input_dim]
    (junction 1450) -> (junction 1433) : {j++;}
    (junction 1433) -> (junction 1413)
    (junction 1448) -> (junction 1450) : {Output_Value[i][j] = Input_Value[i][j];}
    (junction 1413) -> (junction 1442) : {i++;j=0;}
    (junction 1442) -> (junction 1509)
    (junction 1509) -> (junction 1508) : [Input_dim == 1]
    (junction 1509) -> (junction 1431) : {m=Input_dim -1;n = 3;k = 0;}
    (junction 1508) -> (junction 1512)
    (junction 1430) -> (junction 1437) : {temp = 0;n = m-1;}
    (junction 1437) -> (junction 1488) : [n>=0]
    (junction 1488) -> (junction 1474) : [Output_Value[n][k] > Output_Value[m][k]]
    (junction 1454) -> (junction 1430) : [m >= 1]
    (junction 1492) -> (junction 1437) : {n--;}
    (junction 1437) -> (junction 1485)
    (junction 1488) -> (junction 1492)
    (junction 1474) -> (junction 1476) : {temp=Output_Value[n][k]; Output_Value[n][k]=Output_Value[m][k]; Output_Value[m][k]=temp;}
    (junction 1431) -> (junction 1455) : [k<Input_num]
    (junction 1455) -> (junction 1454)
    (junction 1459) -> (junction 1431) : {k++;m=Input_dim -1;}
    (junction 1431) -> (junction 1420)
    (junction 1435) -> (junction 1454) : {m=m-1;}
    (junction 1454) -> (junction 1459)
    (junction 1485) -> (junction 1435)
    (junction 1476) -> (junction 1492)
    (junction 1512) -> (junction 1420)
    (junction 1420) -> (junction 1497) : {h = (Input_dim - 1)/2; k=0;}
    (junction 1497) -> (junction 1499) : [k<Input_num]
    (junction 1499) -> (junction 1501) : {TargetOutput_Value[k] = Output_Value[h][k];}
    (junction 1501) -> (junction 1497) : {k++;}
    (junction 1497) -> (junction 1504)
  (default) -> sort
  data: Input_Value input single; Output_Value output single; Input_dim input uint8; i local uint8; j local uint8; temp local single; k local uint8; n local int8; m local uint8; TargetOutput_Value output single; h local uint8; Input_num input uint8

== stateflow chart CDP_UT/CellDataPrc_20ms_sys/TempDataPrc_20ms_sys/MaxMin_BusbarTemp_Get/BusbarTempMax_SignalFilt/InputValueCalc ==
  state VldValueFilter
    state Default
      Output_Value[0] = Input_Value;
      Output_Value[1] = Input_Value;
      Output_Value[2] = Input_Value;
      Output_Value[3] = Input_Value;
      Output_Value[4] = Input_Value;
    state NotUpdate
      Output_Value[0] = Old_Value[0];
      Output_Value[1] = Old_Value[1];
      Output_Value[2] = Old_Value[2];
      Output_Value[3] = Old_Value[3];
      Output_Value[4] = Old_Value[4];
    state Update
      Output_Value[0] = Input_Value;
      Output_Value[1] = Old_Value[0];
      Output_Value[2] = Old_Value[1];
      Output_Value[3] = Old_Value[2];
      Output_Value[4] = Old_Value[3];
    (default) -> Default
    VldValueFilter -> (junction 1397)
    (junction 1397) -> (junction 1398) : [Rige]
    (junction 1397) -> NotUpdate
    (junction 1398) -> Update
  (default) -> VldValueFilter
  data: Input_Value input single; Rige input boolean; Output_Value output single; Old_Value input single

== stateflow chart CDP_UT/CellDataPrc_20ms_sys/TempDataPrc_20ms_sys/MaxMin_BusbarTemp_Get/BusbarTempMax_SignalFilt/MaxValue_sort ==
  state sort
    (default) -> (junction 1403) : /*Input value sort from big to small*/
    sort -> (junction 1403)
    (junction 1403) -> (junction 1442) : {i = 0;temp = 0;}
    (junction 1442) -> (junction 1433) : [i < Input_dim]
    (junction 1433) -> (junction 1413) : {Output_Value[i] = Input_Value[i];}
    (junction 1413) -> (junction 1442) : {i++;}
    (junction 1442) -> (junction 1431) : {i=0;}
    (junction 1425) -> (junction 1421) : [Output_Value[j] > temp]
    (junction 1431) -> (junction 1430) : [i < Input_dim]
    (junction 1437) -> (junction 1425) : [j < Input_dim]
    (junction 1430) -> (junction 1437) : {temp = 0;Output_index[i] = 0;j = 0;}
    (junction 1425) -> (junction 1404)
    (junction 1421) -> (junction 1418) : {temp = Output_Value[j]; Output_index[i] = j;}
    (junction 1435) -> (junction 1431) : {i++;}
    (junction 1404) -> (junction 1437) : {j++;}
    (junction 1437) -> (junction 1435) : {Output_Value[Output_index[i]] = 0;}
    (junction 1431) -> (junction 1420) : {i= 0;}
    (junction 1418) -> (junction 1404)
    (junction 1420) -> (junction 1426) : [i < Input_dim]
    (junction 1426) -> (junction 1429) : {Output_Value[i] = Input_Value[Output_index[i]];}
    (junction 1429) -> (junction 1420) : {i++;}
    (junction 1420) -> (junction 1438)
  (default) -> sort
  data: Input_Value input single; Output_Value output single; Input_dim input uint8; Output_index output uint8; i local uint8; j local uint8; temp local single

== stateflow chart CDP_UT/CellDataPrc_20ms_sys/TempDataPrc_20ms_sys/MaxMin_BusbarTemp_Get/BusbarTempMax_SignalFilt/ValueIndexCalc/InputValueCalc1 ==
  state VldValueFilter
    state Default
      Output_Value[0] = Input_Value;
      Output_Value[1] = Input_Value;
      Output_Value[2] = Input_Value;
      Output_Value[3] = Input_Value;
      Output_Value[4] = Input_Value;
    state NotUpdate
      Output_Value[0] = Old_Value[0];
      Output_Value[1] = Old_Value[1];
      Output_Value[2] = Old_Value[2];
      Output_Value[3] = Old_Value[3];
      Output_Value[4] = Old_Value[4];
    state Update
      Output_Value[0] = Input_Value;
      Output_Value[1] = Old_Value[0];
      Output_Value[2] = Old_Value[1];
      Output_Value[3] = Old_Value[2];
      Output_Value[4] = Old_Value[3];
    (default) -> Default
    VldValueFilter -> (junction 1397)
    (junction 1397) -> (junction 1398) : [Rige]
    (junction 1397) -> NotUpdate
    (junction 1398) -> Update
  (default) -> VldValueFilter
  data: Input_Value input uint8; Rige input boolean; Output_Value output uint8; Old_Value input uint8

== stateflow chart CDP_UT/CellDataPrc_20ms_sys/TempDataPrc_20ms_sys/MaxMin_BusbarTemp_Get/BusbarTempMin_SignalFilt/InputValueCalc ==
  state VldValueFilter
    state Default
      Output_Value[0] = Input_Value;
      Output_Value[1] = Input_Value;
      Output_Value[2] = Input_Value;
      Output_Value[3] = Input_Value;
      Output_Value[4] = Input_Value;
    state NotUpdate
      Output_Value[0] = Old_Value[0];
      Output_Value[1] = Old_Value[1];
      Output_Value[2] = Old_Value[2];
      Output_Value[3] = Old_Value[3];
      Output_Value[4] = Old_Value[4];
    state Update
      Output_Value[0] = Input_Value;
      Output_Value[1] = Old_Value[0];
      Output_Value[2] = Old_Value[1];
      Output_Value[3] = Old_Value[2];
      Output_Value[4] = Old_Value[3];
    (default) -> Default
    VldValueFilter -> (junction 1397)
    (junction 1397) -> (junction 1398) : [Rige]
    (junction 1397) -> NotUpdate
    (junction 1398) -> Update
  (default) -> VldValueFilter
  data: Input_Value input single; Rige input boolean; Output_Value output single; Old_Value input single

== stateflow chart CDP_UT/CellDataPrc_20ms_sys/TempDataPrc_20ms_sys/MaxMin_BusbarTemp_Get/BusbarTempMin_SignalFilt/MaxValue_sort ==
  state sort
    (default) -> (junction 1403) : /*Input value sort from big to small*/
    sort -> (junction 1403)
    (junction 1403) -> (junction 1442) : {i = 0;temp = 0;}
    (junction 1442) -> (junction 1433) : [i < Input_dim]
    (junction 1433) -> (junction 1413) : {Output_Value[i] = Input_Value[i];}
    (junction 1413) -> (junction 1442) : {i++;}
    (junction 1442) -> (junction 1431) : {i=0;}
    (junction 1425) -> (junction 1421) : [Output_Value[j] > temp]
    (junction 1431) -> (junction 1430) : [i < Input_dim]
    (junction 1437) -> (junction 1425) : [j < Input_dim]
    (junction 1430) -> (junction 1437) : {temp = 0;Output_index[i] = 0;j = 0;}
    (junction 1425) -> (junction 1404)
    (junction 1421) -> (junction 1418) : {temp = Output_Value[j]; Output_index[i] = j;}
    (junction 1435) -> (junction 1431) : {i++;}
    (junction 1404) -> (junction 1437) : {j++;}
    (junction 1437) -> (junction 1435) : {Output_Value[Output_index[i]] = 0;}
    (junction 1431) -> (junction 1420) : {i= 0;}
    (junction 1418) -> (junction 1404)
    (junction 1420) -> (junction 1426) : [i < Input_dim]
    (junction 1426) -> (junction 1429) : {Output_Value[i] = Input_Value[Output_index[i]];}
    (junction 1429) -> (junction 1420) : {i++;}
    (junction 1420) -> (junction 1438)
  (default) -> sort
  data: Input_Value input single; Output_Value output single; Input_dim input uint8; Output_index output uint8; i local uint8; j local uint8; temp local single

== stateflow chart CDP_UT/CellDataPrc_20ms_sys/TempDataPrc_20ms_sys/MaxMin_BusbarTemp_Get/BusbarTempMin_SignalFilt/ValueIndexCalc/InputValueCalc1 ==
  state VldValueFilter
    state Default
      Output_Value[0] = Input_Value;
      Output_Value[1] = Input_Value;
      Output_Value[2] = Input_Value;
      Output_Value[3] = Input_Value;
      Output_Value[4] = Input_Value;
    state NotUpdate
      Output_Value[0] = Old_Value[0];
      Output_Value[1] = Old_Value[1];
      Output_Value[2] = Old_Value[2];
      Output_Value[3] = Old_Value[3];
      Output_Value[4] = Old_Value[4];
    state Update
      Output_Value[0] = Input_Value;
      Output_Value[1] = Old_Value[0];
      Output_Value[2] = Old_Value[1];
      Output_Value[3] = Old_Value[2];
      Output_Value[4] = Old_Value[3];
    (default) -> Default
    VldValueFilter -> (junction 1397)
    (junction 1397) -> (junction 1398) : [Rige]
    (junction 1397) -> NotUpdate
    (junction 1398) -> Update
  (default) -> VldValueFilter
  data: Input_Value input uint8; Rige input boolean; Output_Value output uint8; Old_Value input uint8
